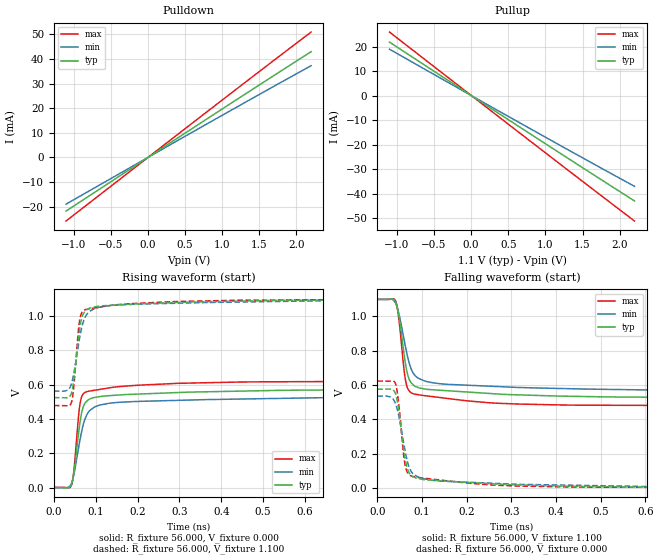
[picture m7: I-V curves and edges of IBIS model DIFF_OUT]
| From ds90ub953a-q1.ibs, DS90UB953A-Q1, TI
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|   DIFF_OUT Model
[Model]   DIFF_OUT
Model_type   Output
Polarity   Non-Inverting
Vmeas = 0.55
Vref = 0
Cref = 0.01pF
Rref = 100000
|   typ   min   max
C_comp   0.1637pF   0.1565pF   0.171pF
|C_comp_pulldown   0.1637pF   0.1565pF   0.171pF
|C_comp_pullup   0.1637pF   0.1561pF   0.1713pF
| Where Nom  PVT is Nominal Process, 1.1V, 27C
|   Fast PVT is Strong Process,  1.101V, -40C
|   Slow PVT is Weak Process,   1.099V, 105C
[Voltage Range]   1.1   1.099   1.101
|Junction Temperature
[Temperature Range]   27   105   -40
[Pullup Reference]   1.1   1.099   1.101
[Pulldown Reference]   0   0   0
[Power Clamp Reference]   1.1   1.099   1.101
[GND Clamp Reference]   0   0   0
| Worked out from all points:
|   slope of the pulldown table from 0 to 0.165 V, typ, clamps not added: 50.6 ohm
|   slope of the pullup table from 0 to 0.165 V, typ, clamps not added: 50.6 ohm
|   falling waveform, R_fixture 56.000, V_fixture 1.100: 20-80 % time 21ps typ, 29.8ps min, 16.5ps max; typ from 1.1 V to 0.524 V
|   rising waveform, R_fixture 56.000, V_fixture 0.000: 20-80 % time 19.4ps typ, 29.4ps min, 14.4ps max; typ from 0.002 V to 0.576 V
|   rising waveform, R_fixture 56.000, V_fixture 1.100: 20-80 % time 18.1ps typ, 26.4ps min, 13.6ps max; typ from 0.524 V to 1.1 V
|   falling waveform, R_fixture 56.000, V_fixture 0.000: 20-80 % time 19.2ps typ, 26.3ps min, 15.3ps max; typ from 0.576 V to 0.002 V
[Pulldown]
|   Voltage   I(typ)   I(min)   I(max)
-1.1V     -21.84mA   -19.02mA   -25.88mA
875.3mV   17.18mA    14.94mA    20.35mA
1.601V    31.38mA    27.26mA    37.2mA
2.2V      42.97mA    37.28mA    50.97mA
[Pullup]
|   Voltage   I(typ)   I(min)   I(max)
-1.1V     21.88mA    18.98mA    25.98mA
743.3mV   -14.59mA   -12.61mA   -17.34mA
1.601V    -31.39mA   -27.08mA   -37.35mA
2.2V      -43.01mA   -37.04mA   -51.21mA
[Ramp]
R_load = 56
|   typ   min   max
dV/dt_r   0.333801/1.93688e-11   0.309597/2.93547e-11   0.361862/1.4424e-11
dV/dt_f   0.334038/2.10412e-11   0.310807/2.97877e-11   0.361312/1.64561e-11
[Falling Waveform]
R_fixture = 56.000
V_fixture = 1.100
V_fixture_min = 1.100
V_fixture_max = 1.100
C_fixture = 0.000
|  time   V(typ)   V(min)   V(max)
0s        1.098V     1.098V     1.098V
40.52ps   1.087V     1.078V     1.092V
47.43ps   1.017V     1.026V     1.006V
60.24ps   778mV      863.2mV    683.7mV
66.26ps   681.3mV    786.5mV    594.3mV
78.11ps   607.6mV    680.9mV    552mV
98.91ps   580.4mV    631.5mV    540.5mV
154.2ps   567.2mV    604.3mV    522.8mV
415.3ps   535.2mV    579.4mV    483.7mV
1.83ns    524.4mV    562.6mV    478.5mV
[Rising Waveform]
R_fixture = 56.000
V_fixture = 0.000
V_fixture_min = 0.000
V_fixture_max = 0.000
C_fixture = 0.000
|  time   V(typ)   V(min)   V(max)
0s        1.915mV    1.766mV    2.302mV
30.62ps   171.8uV    197.6uV    1.81mV
43.22ps   26.44mV    33.45mV    23.69mV
49.11ps   107mV      92.93mV    129.9mV
61.36ps   360.5mV    263.7mV    467mV
68.88ps   459.3mV    353.4mV    541.5mV
85.95ps   516.6mV    449.6mV    562.5mV
135.7ps   536.3mV    492.6mV    582.5mV
445ps     562.1mV    516.1mV    615.1mV
1.83ns    575.6mV    535.2mV    623.1mV
[Rising Waveform]
R_fixture = 56.000
V_fixture = 1.100
V_fixture_min = 1.100
V_fixture_max = 1.100
C_fixture = 0.000
|  time   V(typ)   V(min)   V(max)
0s        524.4mV    562.6mV    478.5mV
29.02ps   523.5mV    564mV      477.4mV
41.88ps   548.6mV    603.1mV    494.4mV
48.25ps   635.6mV    671.2mV    603mV
59.24ps   877.5mV    835.1mV    927.8mV
66.26ps   980.4mV    926.9mV    1.016V
83.17ps   1.042V     1.021V     1.04V
127.7ps   1.06V      1.057V     1.057V
445ps     1.085V     1.08V      1.091V
1.83ns    1.098V     1.098V     1.098V
[Falling Waveform]
R_fixture = 56.000
V_fixture = 0.000
V_fixture_min = 0.000
V_fixture_max = 0.000
C_fixture = 0.000
|  time   V(typ)   V(min)   V(max)
0s        575.6mV    535.2mV    623.1mV
27.95ps   576.4mV    532.1mV    623mV
40.52ps   553.2mV    494.3mV    611.4mV
47.43ps   470mV      430.3mV    508.9mV
58.31ps   248.7mV    276.2mV    213mV
63.77ps   152.5mV    199.2mV    118.3mV
75.87ps   76.92mV    97.6mV     71.22mV
91.58ps   55.34mV    65.25mV    61.94mV
415.3ps   11.71mV    17.95mV    7.176mV
1.83ns    1.915mV    1.766mV    2.302mV
